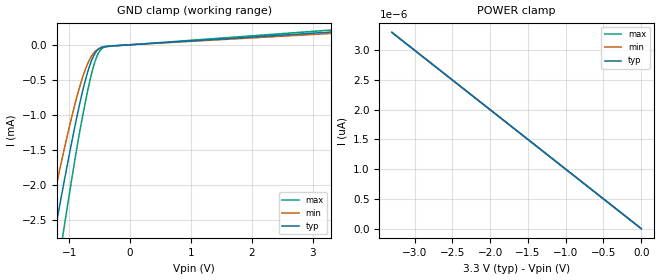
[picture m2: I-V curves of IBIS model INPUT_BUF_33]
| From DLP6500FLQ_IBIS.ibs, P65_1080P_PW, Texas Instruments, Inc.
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[Model]   INPUT_BUF_33
Model_type  Input
Vinl=0.70
Vinh=2.00
| variable   typ   min   max
C_comp   0.33pF   0.28pF   0.42pF
[Temperature Range]   40   140   -40
| Ambient temperature   25   125   -40
[Voltage range]   3.3   3   3.6
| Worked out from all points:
|   GND clamp passes 1 mA (typ) near -0.87 V on its own axis
[GND Clamp]
| INPUT_BUF_33
|   Voltage   I(typ)   I(min)   I(max)
-3.3V     -13.38mA   -11.69mA   -15.85mA
-1.37V    -3.336mA   -2.683mA   -4.25mA
-1.255V   -2.776mA   -2.197mA   -3.588mA
-1.22V    -2.607mA   -2.053mA   -3.389mA
-1.09V    -1.993mA   -1.53mA    -2.655mA
-905mV    -1.167mA   -850.8uA   -1.643mA
-740mV    -529.2uA   -368.3uA   -847.5uA
-605mV    -172.8uA   -128uA     -326.6uA
-500mV    -52.57uA   -49.54uA   -91.53uA
-425mV    -28.52uA   -28.24uA   -37.31uA
-280mV    -15.59uA   -14.16uA   -17.96uA
3.3V      182.1uA    161.7uA    210.3uA
[POWER Clamp]
| INPUT_BUF_33
|   Voltage   I(typ)   I(min)   I(max)
-3.3V     3.3pA      3.3pA      3.3pA
-1.005V   1.005pA    1.005pA    1.005pA
-1V       1pA        999.9fA    1pA
-48.03fV  0A         0A         0A
